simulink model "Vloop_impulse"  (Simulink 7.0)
settings: Solver=ode45  StartTime=0.0  StopTime=1e-2  RelTol=1e-3  AbsTol=1e-6
undefined symbols (not defined in the file or in its folder): plecs
libraries: plecslib_extras2 x1

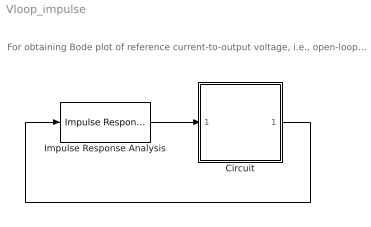
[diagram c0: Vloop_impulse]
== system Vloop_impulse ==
  note: For obtaining Bode plot of reference current-to-output voltage, i.e., open-loop voltage control transfer function.
  Circuit : Subsystem  LoadFcn=plecs('sl', 200);  InitFcn=plecs('sl', 214);  StartFcn=plecs('sl', 208);  StopFcn=plecs('sl', 209);  mask(PlecsCircuit){PLECSData=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}
      mask prompts: PLECSData "PLECS Data (Do not delete or modify!)"
      mask init:
      | % PLACE CUSTOM INITIALIZATIONS ABOVE
      | % DO NOT REMOVE
      | plecs('sl', 215);
      | % DO NOT REMOVE
  Impulse Response Analysis : plecslib_extras2/Analysis Tools/Impulse Response Analysis  SystemSampleTime=-1  FreqRange=[0.1 1e3]  FreqScale=logarithmic  NPoints=101  Perturbation=1e-4  Compensation=discrete pulse  TimeSpan=1/50e3  TStart=0  MaxIter=20  Tolerance=1e-5  Display=iteration  HideScopes=on  HiddenStates=error  OutputName=Vconverter  BodePlot=on  JPert=1e-4  NInitCycles=10
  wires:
  Impulse Response Analysis/1 -> Circuit/1(pert)
  Circuit/1(vo) -> Impulse Response Analysis/1

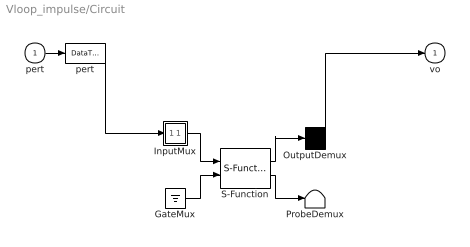
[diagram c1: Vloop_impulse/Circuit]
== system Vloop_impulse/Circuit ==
  pert : Inport  PortDimensions=1  OutDataType=sfix(16)  OutScaling=2^0
  " GateMux " : Ground
  " InputMux " : Subsystem
  " OutputDemux " : Demux  Outputs=[ 1 ]
  " ProbeDemux " : Terminator
  " S-Function " : S-Function  FunctionName=plecs
  " pert " : DataTypeConversion
  vo : Outport  PortDimensions=1  OutDataType=sfix(16)  OutScaling=2^0
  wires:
  " S-Function "/1 -> " OutputDemux "/1
  " InputMux "/1(Out) -> " S-Function "/1
  " GateMux "/1 -> " S-Function "/2
  " S-Function "/2 -> " ProbeDemux "/1
  pert/1 -> " pert "/1
  " pert "/1 -> " InputMux "/1(In1)
  " OutputDemux "/1 -> vo/1

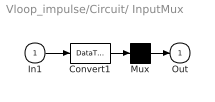
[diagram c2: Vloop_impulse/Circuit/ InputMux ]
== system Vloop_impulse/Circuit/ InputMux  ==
  In1 : Inport  OutDataType=sfix(16)  OutScaling=2^0
  Convert1 : DataTypeConversion  OutDataType=sfix(16)  OutScaling=2^0
  Mux : Mux  Inputs=[ 1 ]
  Out : Outport  OutDataType=sfix(16)  OutScaling=2^0
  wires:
  Mux/1 -> Out/1
  In1/1 -> Convert1/1
  Convert1/1 -> Mux/1
